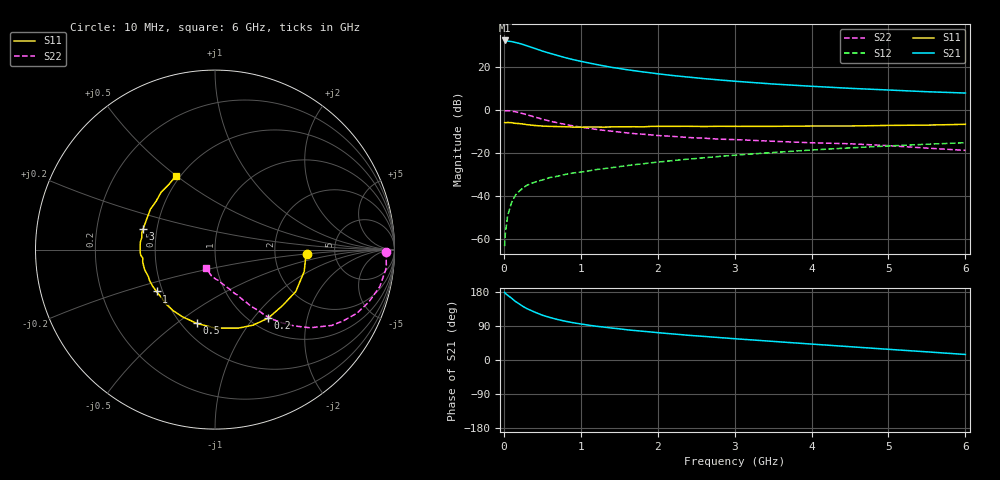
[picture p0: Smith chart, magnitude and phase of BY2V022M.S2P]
! SIEMENS Small Signal Semiconductors
! BFY420
! Si NPN RF SIEGET Grounded Emitter Transistor in MICRO-X
! VCE = 2 V  IC = 22 mA
! Common Emitter S-Parameters:  October  1996
# GHz  S  MA  R  50
!  f  S11  S21  S12  S22
! GHz  MAG  ANG  MAG  ANG  MAG  ANG  MAG  ANG
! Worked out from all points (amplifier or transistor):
!   36 points, 10 MHz to 6 GHz, reference 50 ohm
!   highest |S21| = 32.2 dB at 10 MHz (marker M1)
!   |S21| within 3 dB of that: start of sweep to 344.6 MHz
!   unconditionally stable (mu >= 1): 1.782 GHz to end of sweep
!   at 250 MHz: K = 0.30, MSG = 33.2 dB, |S12| = -36.1 dB
!   at 1.4 GHz: K = 0.93, MSG = 23.2 dB, |S12| = -26.7 dB
!   at 6 GHz: K = 1.07, MAG = 9.8 dB, |S12| = -15.2 dB
!   S11 on the Smith chart (normalised r, x): 10 MHz: 3.07, -0.22; 200 MHz: 1.20, -1.19; 500 MHz: 0.59, -0.59; 1 GHz: 0.46, -0.26; 3 GHz: 0.42, +0.12; 6 GHz: 0.47, +0.50
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0.01  0.5113 -3.0  40.67 178.5  0.0007 117.0  0.9548 -0.7
0.02  0.507 -5.5  40.25 175.6  0.0014 86.5  0.9539 -2.0
0.05  0.5118 -13.7  39.27 170.8  0.0036 83.9  0.9603 -6.0
0.1  0.5072 -27.4  38.35 163.2  0.0071 82.2  0.9409 -12.7
0.15  0.4887 -39.7  36.57 154.5  0.0106 73.9  0.9057 -18.8
0.2  0.4834 -52.2  34.83 148.0  0.0131 72.0  0.8669 -24.1
0.25  0.4714 -63.3  32.74 141.2  0.0157 69.0  0.819 -28.9
0.3  0.4567 -73.1  30.61 135.6  0.018 65.1  0.7757 -33.0
0.4  0.4371 -90.1  26.69 126.5  0.0213 61.9  0.6861 -39.4
0.5  0.4235 -103.9  23.14 118.3  0.0239 59.7  0.6121 -44.0
0.6  0.4158 -115.9  20.46 112.1  0.0272 58.2  0.5518 -47.6
0.7  0.4124 -124.2  18.23 106.8  0.0292 58.7  0.5028 -50.5
0.8  0.4083 -132.4  16.24 102.3  0.0321 56.7  0.4612 -52.7
1  0.4006 -144.4  13.38 95.1  0.0364 57.3  0.4007 -55.6
1.1  0.403 -149.8  12.3 92.0  0.0387 57.8  0.3764 -57.4
1.6  0.4079 -167.7  8.552 79.8  0.0514 57.4  0.2942 -63.0
2.2  0.4176 178.2  6.256 68.7  0.0673 55.9  0.2442 -68.7
3  0.4165 164.0  4.629 56.2  0.0896 51.9  0.2059 -75.1
3.5  0.417 155.6  3.987 49.1  0.1033 48.5  0.1882 -79.5
4.5  0.4245 140.6  3.168 35.1  0.1323 40.2  0.1648 -88.4
5.5  0.4453 125.0  2.642 21.5  0.1607 30.9  0.1307 -104.8
6  0.4649 118.1  2.464 14.6  0.1741 26.0  0.1158 -116.9
